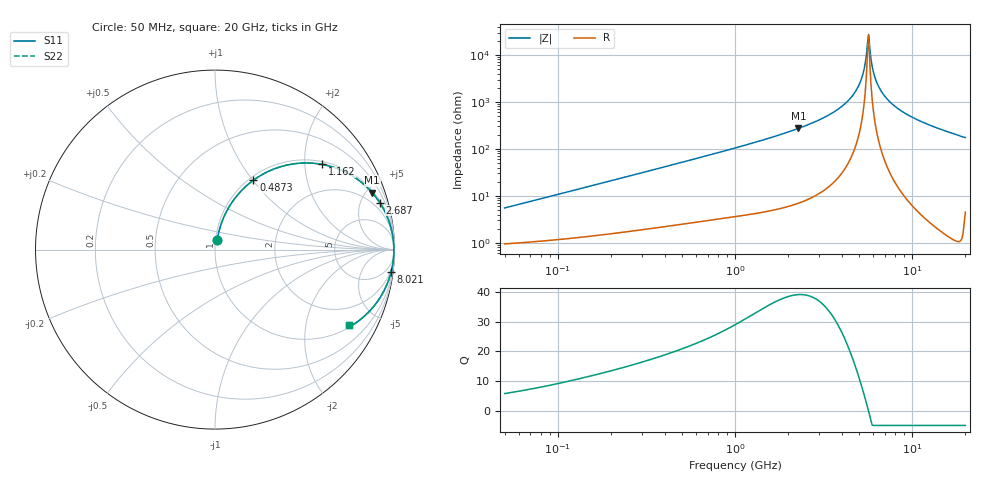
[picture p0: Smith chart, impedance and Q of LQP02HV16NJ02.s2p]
!Murata Part Number: LQP02HV16NJ02
!These Parameters are Measured in Series Mode Connection
!  o--[Z]--o
!Port1  Port2
!  o-------o
!Freq. Start=50[MHz] Stop=20[GHz], 401[Steps]
# Hz S RI R 50
!Freq.(Hz) S11(Real) S11(Imag) S21(Real) S21(Imag) S12(Real) S12(Imag) S22(Real) S22(Imag)
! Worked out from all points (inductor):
!   401 points, 50 MHz to 20 GHz, reference 50 ohm
!   read as one part in series: L = 17.2 nH near 51.52 MHz
!   highest Q = 39.1 at 2.279 GHz (marker M1), where L = 19 nH
!   self-resonance near 5.599 GHz
!   S11 on the Smith chart (normalised r, x): 50 MHz: 1.02, +0.11; 487.3 MHz: 1.05, +1.01; 1.162 GHz: 1.08, +2.45; 2.687 GHz: 1.18, +6.94; 8.021 GHz: 1, -16; 20 GHz: 1.09, -3.50
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5e7  0.0123 0.0533  0.9877 -0.0533  0.9877 -0.0533  0.0123 0.0533
1.364002e8  0.0327 0.1381  0.9673 -0.1381  0.9673 -0.1381  0.0327 0.1381
3.721004e8  0.143 0.3236  0.857 -0.3236  0.857 -0.3236  0.143 0.3236
4.872511e8  0.2137 0.3863  0.7863 -0.3863  0.7863 -0.3863  0.2137 0.3863
1e9  0.5207 0.4826  0.4793 -0.4826  0.4793 -0.4826  0.5207 0.4826
1.161586e9  0.5964 0.4748  0.4036 -0.4748  0.4036 -0.4748  0.5964 0.4748
2.279204e9  0.8752 0.318  0.1248 -0.318  0.1248 -0.318  0.8752 0.318
2.687447e9  0.9177 0.2622  0.0823 -0.2622  0.0823 -0.2622  0.9177 0.2622
2.728004e9  0.921 0.257  0.079 -0.257  0.079 -0.257  0.921 0.257
3.736399e9  0.9729 0.1464  0.0271 -0.1464  0.0271 -0.1464  0.9729 0.1464
4.608136e9  0.9905 0.0726  0.00946 -0.0726  0.00946 -0.0726  0.9905 0.0726
5.194772e9  0.9953 0.0306  0.00471 -0.0306  0.00471 -0.0306  0.9953 0.0306
5.352748e9  0.9959 0.0201  0.00409 -0.0201  0.00409 -0.0201  0.9959 0.0201
5.515528e9  0.9963 0.00959  0.0037 -0.00959  0.0037 -0.00959  0.9963 0.00959
5.683258e9  0.9965 -0.000897  0.00354 0.000897  0.00354 0.000897  0.9965 -0.000897
5.769027e9  0.9965 -0.00614  0.00354 0.00614  0.00354 0.00614  0.9965 -0.00614
6.034176e9  0.9961 -0.0219  0.00389 0.0219  0.00389 0.0219  0.9961 -0.0219
6.311513e9  0.9953 -0.0377  0.00475 0.0377  0.00475 0.0377  0.9953 -0.0377
7.442007e9  0.9877 -0.0957  0.0123 0.0957  0.0123 0.0957  0.9877 -0.0957
8.020766e9  0.9818 -0.1223  0.0182 0.1223  0.0182 0.1223  0.9818 -0.1223
1.166392e10  0.9265 -0.2562  0.0735 0.2562  0.0735 0.2562  0.9265 -0.2562
2e10  0.748 -0.4215  0.252 0.4215  0.252 0.4215  0.748 -0.4215
